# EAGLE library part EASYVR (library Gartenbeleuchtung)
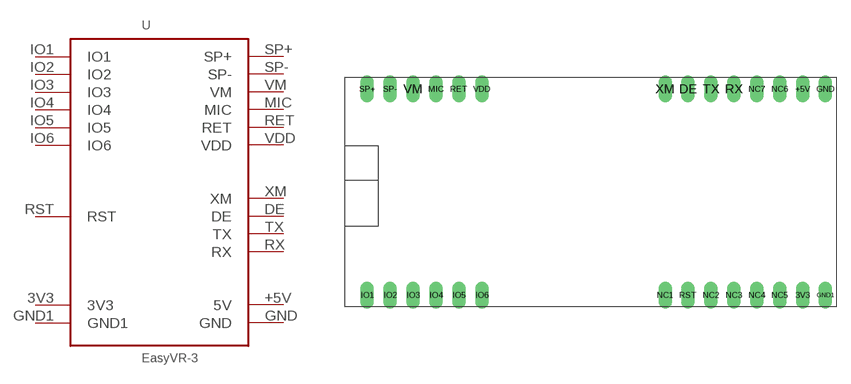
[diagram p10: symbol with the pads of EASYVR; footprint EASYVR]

Designator prefix -

## EASYVR  [EASYVR]
3V3  3V3  pwr
+5V  5V  pwr
DE  DE
GND  GND  pwr
GND1  GND1  pwr
IO1  IO1
IO2  IO2
IO3  IO3
IO4  IO4
IO5  IO5
IO6  IO6
MIC  MIC
RET  RET
RST  RST
RX  RX
SP+  SP+
SP-  SP-
TX  TX
VDD  VDD
VM  VM
XM  XM

## Footprint EASYVR (pad centres in mm)
drill 1 pad 1.422 long: 3V3 48.26,0; +5V 48.26,22.86; DE 35.56,22.86; GND 50.8,22.86; GND1 50.8,0; IO1 0,0; IO2 2.54,0; IO3 5.08,0; IO4 7.62,0; IO5 10.16,0; IO6 12.7,0; MIC 7.62,22.86; NC1 33.02,0; NC2 38.1,0; NC3 40.64,0; NC4 43.18,0; NC5 45.72,0; NC6 45.72,22.86; NC7 43.18,22.86; RET 10.16,22.86; RST 35.56,0; RX 40.64,22.86; SP+ 0,22.86; SP- 2.54,22.86; TX 38.1,22.86; VDD 12.7,22.86; VM 5.08,22.86; XM 33.02,22.86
